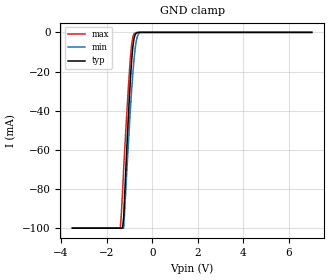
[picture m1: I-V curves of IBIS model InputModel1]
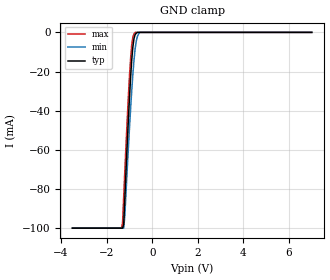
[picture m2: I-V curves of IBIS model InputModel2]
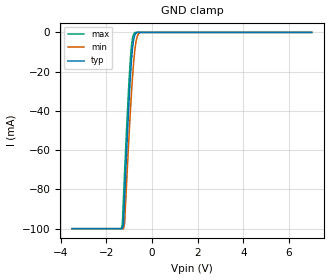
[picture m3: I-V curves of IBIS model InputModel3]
[IBIS Ver]   2.1
[File name]   e_200bl3.ibs   | e_= TSOP, f200bl= abbr chip name, 3= 3.3V Vcc
[File Rev]   2.00
[Date]   13-March-1996
[Source]   File generated from lab measurements at Intel Corporation
[Notes]   Rev 2.00 All data was replaced by actual measurements
   performed in a lab.
[Disclaimer] INTEL DEVELOPER'S SOFTWARE LICENSE AGREEMENT
| BY USING THIS SOFTWARE, YOU ARE AGREEING TO BE BOUND
| BY THE TERMS OFTHIS AGREEMENT.  DO NOT USE THE SOFTWARE
| UNTIL YOU HAVE CAREFULLY READAND AGREED TO THE FOLLOWING
| TERMS AND CONDITIONS.  IF YOU DO NOT AGREETO THE TERMS
| OF THIS AGREEMENT, PROMPTLY RETURN THE SOFTWARE PACKAGE
| ANDANY ACCOMPANYING ITEMS.
| IF YOU USE THIS SOFTWARE, YOU WILL BE BOUND BY THE TERMS
| OF THIS AGREEMENT
| LICENSE: Intel Corporation ("Intel") grants you the non-exclusive right
| to use the enclosed software program ("Software").  You will not use,
| copy, modify, rent, sell or transfer the Software or any portion
| thereof, except as provided in this Agreement.
| System OEM Developers may:
| 1.   Copy the Software for support, backup or archival purposes;
| 2.   Install, use, or distribute Intel owned Software in object code
|   only;
| 3.   Modify and/or use Software source code that Intel directly makes
|   available to you as an OEM Developer;
| 4.   Install, use, modify, distribute, and/or make or have made
|   derivatives ("Derivatives") of Intel owned Software under the
|   terms and conditions in this Agreement, ONLY if you are a System
|   OEM Developer and NOT an end-user.
| RESTRICTIONS:
| YOU WILL NOT:
| 1.   Copy the Software, in whole or in part, except as provided for
|   in this Agreement;
| 2.   Decompile or reverse engineer any Software provided in object
|   code format;
| 3.   Distribute any Software or Derivative code to any end-users,
|   unless approved by Intel in a prior writing.
| TRANSFER: You may transfer the Software to another OEM
| Developer if thereceiving party agrees to the terms of this
| Agreement at the sole risk of any receiving party.
| OWNERSHIP AND COPYRIGHT OF SOFTWARE:
| Title to the Software and all copies thereof remain with Intel
| or its vendors.  The Software iscopyrighted and is protected by
| United States and international copyright laws.  You will not
| remove the copyright notice from the Software.  You agree to
| prevent any unauthorized copying of the Software.
| DERIVATIVE WORK: OEM Developers that make or have made
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[Copyright]   Copyright 1996, Intel Corporation, All Rights Reserved
[Component]   E28F200BL   | 56-lead TSOP package, 28F200BL
[Manufacturer]  Intel   | Boot Block (tm)
|   | operating in 3.3V Vcc range
[Package]
| Variable   typ   min   max
|The following values apply for the Copper leadframe.
R_pkg   48m   41m   54m
L_pkg   4.92nH   4.44nH   5.39nH
C_pkg   0.48pF   0.45pF   0.50pF
|The following values apply for the Alloy-42 leadframe.
|R_pkg   195m   180m   210m
|L_pkg   4.92nH   4.44nH   5.39nH
|C_pkg   0.48pF   0.45pF   0.50pF
|*****************************Pin Definitions**********************************
[Pin]   signal_name   model_name   R_pin   L_pin   C_pin
 1   NC   InputModel6
 2   NC   InputModel6
 3   A15   InputModel1
 4   A14   InputModel1
 5   A13   InputModel1
 6   A12   InputModel1
 7   A11   InputModel1
 8   A10   InputModel1
 9   A09   InputModel1
10   A08   InputModel1
11   NC   InputModel6
12   NC   InputModel6
13   WE#   InputModel5
14   RP#   InputModel3
15   NC   InputModel6
16   NC   InputModel6
17   VPP   POWER
18   DU   InputModel6
19   NC   InputModel6
20   NC   InputModel1
21   A07   InputModel1
22   A06   InputModel1
23   A05   InputModel1
24   A04   InputModel1
25   A03   InputModel1
26   A02   InputModel1
27   A01   InputModel1
28   NC   InputModel6
29   NC   InputModel6
30   NC   InputModel6
31   A0   InputModel2
32   CE#   InputModel2
33   GND   GND
34   OE#   InputModel4
35   DQ0   InputOutput1
36   DQ8   InputOutput1
37   DQ1   InputOutput1
38   DQ9   InputOutput1
39   DQ2   InputOutput1
40   DQ10   InputOutput1
41   DQ3   InputOutput1
42   DQ11   InputOutput1
43   VCC   POWER
44   VCC   POWER
45   DQ4   InputOutput1
46   DQ12   InputOutput1
47   DQ5   InputOutput1
48   DQ13   InputOutput1
49   DQ6   InputOutput1
50   DQ14   InputOutput1
51   DQ7   InputOutput1
52   DQ15   InputOutput2
53   GND   GND
54   BYTE#   InputModel2
55   A16   InputModel2
56   NC   InputModel6
|***********************Input Model 6******************************
[Model]   InputModel6
Model_type   Input
|   Model for DU and NC pins, excluding Pin #20.
Vinl = 0.8V
Vinh = 2.0V
|Variable   Typ   Min   Max
C_comp   5.61p   NA   7.6p
[Voltage Range]   3.3V   3.0V   3.6V
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| Models and submodels in the file (8): InputModel1 (Input), InputModel2 (Input), InputModel3 (Input), InputModel4 (Input), InputModel5 (Input), InputModel6 (Input), InputOutput1 (I/O), InputOutput2 (I/O)
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|*********************Input Model 1************************************
[Model]   InputModel1
Model_type   Input
|   Model for A[15:1] & NC (pin 20).
Vinl = 0.8V
Vinh = 2.0V
|Variable   Typ   Min   Max
C_comp   5.61p   NA   7.6p
[Voltage Range]   3.3V   3.0V   3.6V
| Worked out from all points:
|   GND clamp passes 1 mA (typ) near -0.74 V on its own axis
[GND_clamp]
|Voltage  I(typ)   I(min)   I(max)
-3.5V     -100mA     -100mA     -100mA
-1.4V     -100mA     -100mA     -100mA
-1.35V    -100mA     -100mA     -92.06mA
-1.3V     -100mA     -100mA     -81.04mA
-1.25V    -94.05mA   -100mA     -69.23mA
-1.1V     -55.84mA   -68.26mA   -38.39mA
-1V       -32.84mA   -47.78mA   -19.9mA
-900mV    -13.97mA   -29.09mA   -6.016mA
-800mV    -3.185mA   -14.07mA   -792.3uA
-700mV    -426.8uA   -4.481mA   0A
-550mV    0A         0A         0A
7V        0A         0A         0A
[Power_clamp]
| Input buffer circuits of this product do not intrinsically
| require a [Power_clamp] definition.  This zero current
| [Power_clamp] table is provided for the compatibility with
| some IBIS parsers.
|Voltage  I(typ)   I(min)   I(max)
-3.3V     0A         0A         0A
0V        0A         0A         0A
3.3V      0A         0A         0A
7V        0A         0A         0A
|*********************Input Model 2******************************
[Model]   InputModel2
Model_type   Input
|   Model for A[0], A[16], CE# & BYTE# pins.
Vinl = 0.8V
Vinh = 2.0V
|Variable   Typ   Min   Max
C_comp   5.61p   NA   7.6p
[Voltage Range]   3.3V   3.0V   3.6V
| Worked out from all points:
|   GND clamp passes 1 mA (typ) near -0.74 V on its own axis
[GND_clamp]
|Voltage  I(typ)   I(min)   I(max)
-3.5V     -100mA     -100mA     -100mA
-1.35V    -100mA     -100mA     -100mA
-1.3V     -100mA     -100mA     -97.31mA
-1.25V    -97.98mA   -100mA     -83.77mA
-1.2V     -84.29mA   -93.56mA   -70.52mA
-1.05V    -45.71mA   -60.05mA   -33.65mA
-950mV    -23.43mA   -39.44mA   -13.59mA
-850mV    -7.586mA   -21.73mA   -2.468mA
-750mV    -1.17mA    -8.517mA   0A
-650mV    0A         -2.085mA   0A
-550mV    0A         0A         0A
7V        0A         0A         0A
[Power_clamp]
| Input buffer circuits of this product do not intrinsically
| require a [Power_clamp] definition.  This zero current
| [Power_clamp] table is provided for the compatibility with
| some IBIS parsers.
|Voltage  I(typ)   I(min)   I(max)
-3.3V     0A         0A         0A
0V        0A         0A         0A
3.3V      0A         0A         0A
7V        0A         0A         0A
|***********************Input Model 3******************************
[Model]   InputModel3
Model_type   Input
|   Model for RP# pin.
Vinl = 0.8V
Vinh = 2.0V
|Variable   Typ   Min   Max
C_comp   5.61p   NA   7.6p
[Voltage Range]   3.3V   3.0V   3.6V
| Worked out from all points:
|   GND clamp passes 1 mA (typ) near -0.74 V on its own axis
[GND_clamp]
|Voltage  I(typ)   I(min)   I(max)
-3.5V     -100mA     -100mA     -100mA
-1.35V    -100mA     -100mA     -100mA
-1.3V     -100mA     -100mA     -97.77mA
-1.25V    -97.89mA   -100mA     -84.11mA
-1.2V     -84.17mA   -97.43mA   -70.88mA
-1.05V    -45.52mA   -62.23mA   -33.85mA
-950mV    -23.27mA   -40.65mA   -13.74mA
-850mV    -7.538mA   -22.21mA   -2.542mA
-750mV    -1.177mA   -8.633mA   0A
-650mV    0A         -2.115mA   0A
-550mV    0A         0A         0A
7V        0A         0A         0A
[Power_clamp]
| Input buffer circuits of this product do not intrinsically
| require a [Power_clamp] definition.  This zero current
| [Power_clamp] table is provided for the compatibility with
| some IBIS parsers.
|Voltage  I(typ)   I(min)   I(max)
-3.3V     0A         0A         0A
0V        0A         0A         0A
3.3V      0A         0A         0A
7V        0A         0A         0A
